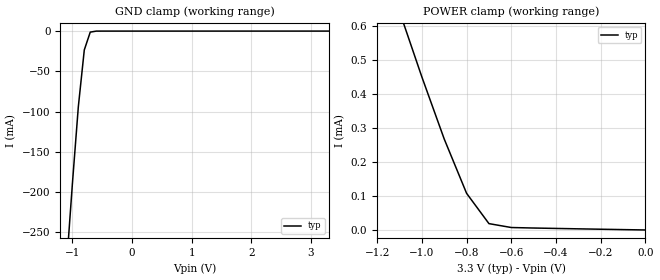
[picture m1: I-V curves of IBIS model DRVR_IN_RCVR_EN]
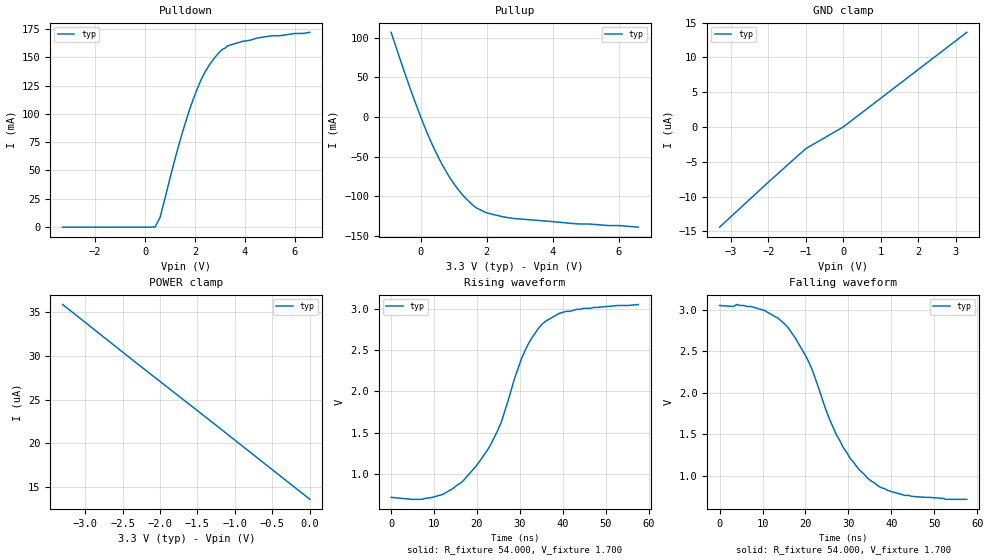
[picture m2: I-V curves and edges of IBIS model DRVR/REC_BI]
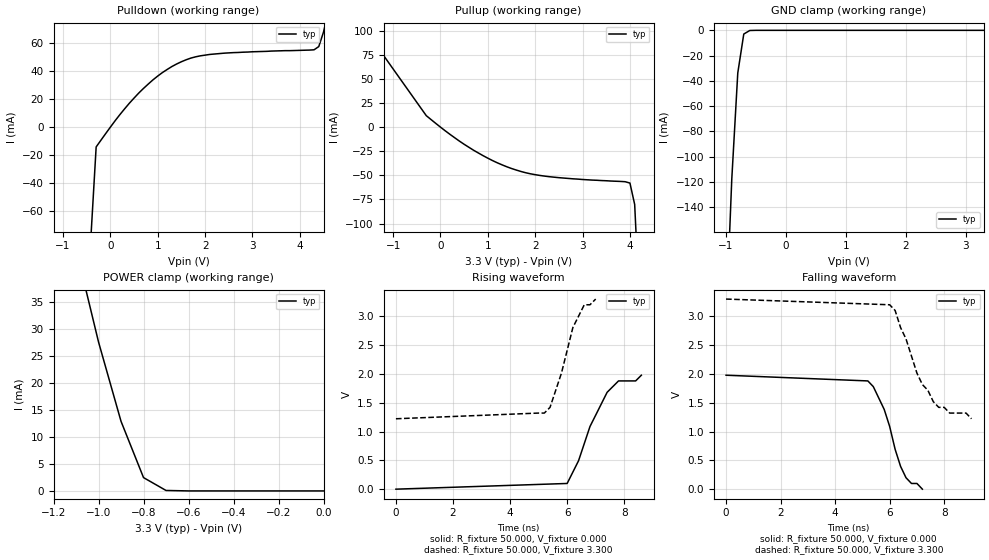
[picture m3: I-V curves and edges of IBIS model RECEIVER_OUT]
|   Texas Instruments Incorporated
|   Data Transmissions Products
|   IBIS Model for SN65HVD11
|   8D SOIC Package
[IBIS Ver]   3.2
[Comment char]   |_char
[File name]   3hvd11.ibs
[File Rev]   1.1
[Date]   11Apr07
[Source]   File originated at Texas Instruments Incorporated.
   Data Transmission Products Group.
[Notes]
[Disclaimer]
(C) Copyright Texas Instruments Incorporated 2002
   All rights reserved
  Texas Instruments Incorporated hereby grants 1the user of this IBIS
model a non-exclusive, nontransferable license to use this IBIS model
under the following terms.  Before using this IBIS model, the user
should read this license.  If the user does not accept these terms,
the IBIS model should be returned to Texas Instruments within 30 days.
  The user is granted this license only to use the IBIS model and
is not granted rights to sell, load, rent, lease or license the IBIS
model in whole or in part, or in modified form to anyone other than
user.  User may modify the IBIS model to suit its specific applications
but rights to derivative works and such modifications shall belong to
Texas Instruments.
  This IBIS model is provided on an "AS IS" basis and Texas Instruments
makes absolutely no warranty with respect to the information contained
herein.  TEXAS INSTRUMENTS DISCLAIMS AND CUSTOMER WAIVES ALL WARRANTIES,
EXPRESS OR IMPLIED, INCLUDING WARRANTIES OF MERCHANTABILITY OR FITNESS
FOR A PARTICULAR PURPOSE. The entire risk as to quality and performance
is with the Customer. ACCORDINGLY, IN NO EVENT SHALL THE COMPANY BE LIABLE
FOR ANY DAMAGES, WHETHER IN CONTRACT OR TORT,INCLUDING ANY LOST PROFITS
OR OTHER INCIDENTAL, CONSEQUENTIAL, EXEMPLARY, OR PUNITIVE DAMAGES ARISING
OUT OF THE USE OR APPLICATION OF THE IBIS model provided in this package.
Further, Texas Instruments reserves the right to discontinue or make changes
without notice to any product herein to improve reliability, function, or
design. Texas Instruments does not convey any license under patent rights
or any other intellectual property rights, including those of third parties.
Contact Texas Instruments at ATTN:DATA TRANSMISSIONS
[Copyright]   Copyright 2002, Texas Instruments, All Rights Reserved
[Component]   HVD11D
[Manufacturer]  Texas Instruments Incorporated
[Package]
|   typ   min   max
R_pkg   0.036   0.033   0.039
L_pkg   3.340nH   2.445nH   4.233nH
C_pkg   0.470pF   0.308pF   0.631pF
[Pin]   signal_name   model_name   R_pin   L_pin   C_pin
1   R   RECEIVER_OUT   0.034   4.233n   0.630p
2   RE   DRVR_IN_RCVR_EN   0.038   2.445n   0.309p
3   DE   DRIVER_EN   0.039   2.448n   0.309p
4   D   DRVR_IN_RCVR_EN   0.033   4.231n   0.631p
5   GND   GND   0.033   4.230n   0.630p
6   A   DRVR/REC_BI   0.039   2.450n   0.308p
7   B   DRVR/REC_BI   0.039   2.448n   0.309p
8   VCC   POWER   0.033   4.231n   0.630p
[Diff_pin]   inv_pin   vdiff   tdelay_typ   tdelay_min   tdelay_max
| The 'A' pin is Diff_pin and the 'B' pin is the inv_pin
6   7   0.200   0 0 0
| Models and submodels in the file (4): DRVR_IN_RCVR_EN (Input), DRIVER_EN (Input), DRVR/REC_BI (I/O), RECEIVER_OUT (3-state)
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|   Driver Input / Receiver Enable Model
[Model]   DRVR_IN_RCVR_EN
Model_type   Input
|Signals   D,RE
Vinh = 2.0
Vinl = 0.8
|   typ   min   max
C_comp   13pF   8pF   16pF
|   typ   min   max
[Temperature Range]   25.0   NA   NA
[Voltage range]   3.3V   3.0V   3.6V
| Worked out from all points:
|   GND clamp passes 1 mA (typ) near -0.68 V on its own axis
|   POWER clamp passes 1 mA (typ) near -1.28 V on its own axis
[GND_clamp]
|   Voltage   I(typ)   I(min)   I(max)
-3.3V     -2.53A     NA         NA
-2V       -1.22A     NA         NA
-1V       -190mA     NA         NA
-900mV    -93.9mA    NA         NA
-800mV    -23.4mA    NA         NA
-700mV    -1.29mA    NA         NA
-600mV    -39.4uA    NA         NA
3.3V      8.15pA     NA         NA
[Power_clamp]
| Note that the[POWER_clamp]voltage table is referenced to Vcc
| and is calculated using Vtable=Vcc - Vmeasured.
|   Voltage   I(typ)   I(min)   I(max)
-3.3V     5.2mA      NA         NA
-1.1V     644uA      NA         NA
-1V       451uA      NA         NA
-900mV    268uA      NA         NA
-800mV    108uA      NA         NA
-700mV    18.7uA     NA         NA
-600mV    7.22uA     NA         NA
0V        8.15pA     NA         NA
|   Driver Output / Receiver Input Model
[Model]   DRVR/REC_BI
Model_type   I/O
| Signals   A,B
Vinl = 0.9V
Vinh = 2.8V
Vmeas = 1.7V   |Reference voltage for timing measurements
Cref = 50pF   |Timing specification test load capacitance value
Rref = 54   |Note: 54 Ohm load; single-ended configuration
|   Timing specification test load voltage
| variable   typ   min   max
C_comp   32pF   26pF   38pF
|   typ   min   max
[Temperature Range]   25.0   NA   NA
[Voltage range]   3.3V   3.0V   3.6V
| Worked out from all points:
|   slope of the pulldown table from 0 to 0.495 V, typ, clamps not added: 120 ohm
|   slope of the pullup table from 0 to 0.495 V, typ, clamps not added: 10.4 ohm
|   rising waveform, R_fixture 54.000, V_fixture 1.700: 20-80 % time 11.1ns typ, NA min, NA max; typ from 0.714 V to 3.05 V
|   falling waveform, R_fixture 54.000, V_fixture 1.700: 20-80 % time 12.4ns typ, NA min, NA max; typ from 3.05 V to 0.714 V
[Pulldown]
|   Voltage   I(typ)   I(min)   I(max)
-3.3V     -26.2uA    NA         NA
400mV     110uA      NA         NA
600mV     8.53mA     NA         NA
1.2V      60.3mA     NA         NA
1.8V      105mA      NA         NA
2.2V      128mA      NA         NA
2.4V      137mA      NA         NA
2.8V      150mA      NA         NA
3.3V      160mA      NA         NA
3.9V      164mA      NA         NA
5.1V      169mA      NA         NA
6.6V      172mA      NA         NA
[Pullup]
|   Voltage   I(typ)   I(min)   I(max)
| Note that the[Pullup]voltage table is referenced to Vcc
| and is calculated using Vtable=Vcc - Vmeasured.
-900mV    107mA      NA         NA
-500mV    57.3mA     NA         NA
-100mV    10.9mA     NA         NA
200mV     -20.7mA    NA         NA
400mV     -39.4mA    NA         NA
700mV     -63.8mA    NA         NA
1V        -83.9mA    NA         NA
1.3V      -99.8mA    NA         NA
1.6V      -112mA     NA         NA
2V        -121mA     NA         NA
2.8V      -128mA     NA         NA
6.6V      -139mA     NA         NA
[GND_clamp]
|   Voltage   I(typ)   I(min)   I(max)
| Outputs in High Impedance (off)
-3.3V     -14.4uA    NA         NA
-2V       -7.94uA    NA         NA
-1V       -3.12uA    NA         NA
0V        -410pA     NA         NA
3.3V      13.6uA     NA         NA
[POWER_clamp]
|   Voltage   I(typ)   I(min)   I(max)
| Note that the [POWER_clamp] voltage table is referenced to Vcc
| and is calculated using Vtable = Vcc - Vmeasured.
| Outputs in Tri-state.
-3.3V     35.9uA     NA         NA
-2.3V     29.1uA     NA         NA
-1.3V     22.4uA     NA         NA
0V        13.6uA     NA         NA
[Ramp]
|   typ   min   max
dV/dt_r   1.188/11.2ns   NA   NA
dV/dt_f   1.200/12.8ns   NA   NA
R_load = 54ohm | Note: The measurement is on a single-ended configuration
|   with 54ohm line-to-line.
[Rising Waveform]
R_fixture = 54.000
V_fixture = 1.700
C_fixture = 0.000
L_fixture = 0.000
|  time   V(typ)   V(min)   V(max)
0s        714mV      NA         NA
7.2ns     690.2mV    NA         NA
12ns      749.6mV    NA         NA
19.2ns    1.058V     NA         NA
22.4ns    1.284V     NA         NA
25.6ns    1.617V     NA         NA
31.2ns    2.496V     NA         NA
36ns      2.852V     NA         NA
43.2ns    2.995V     NA         NA
57.6ns    3.054V     NA         NA
[Falling Waveform]
R_fixture = 54.000
V_fixture = 1.700
C_fixture = 0.000
L_fixture = 0.000
|  time   V(typ)   V(min)   V(max)
0s        3.054V     NA         NA
10.4ns    2.995V     NA         NA
16ns      2.782V     NA         NA
20.8ns    2.369V     NA         NA
25.6ns    1.683V     NA         NA
28.8ns    1.34V      NA         NA
32ns      1.104V     NA         NA
35.2ns    938.6mV    NA         NA
43.2ns    761.3mV    NA         NA
57.6ns    714mV      NA         NA
[Model]   RECEIVER_OUT
Model_type   3-state
| Signals   R
Vmeas = 1.5V   |Reference voltage for timing measurements
Cref = 15pF   |Timing specification test load capacitance value
Vref = 0   |Timing specification test load voltage; GND
| variable   typ   min   max
C_comp   13pF   8pF   16pF
|   typ   min   max
[Temperature Range]   25.0   NA   NA
[Voltage range]   3.3V   3.0V   3.6V
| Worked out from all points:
|   slope of the pulldown table from 0 to 0.495 V, typ, clamps not added: 24.1 ohm
|   slope of the pullup table from 0 to 0.495 V, typ, clamps not added: 28.1 ohm
|   GND clamp passes 1 mA (typ) near -0.63 V on its own axis
|   POWER clamp passes 1 mA (typ) near -0.74 V on its own axis
|   rising waveform, R_fixture 50.000, V_fixture 0.000: 20-80 % time 1ns typ, NA min, NA max; typ from 0 V to 1.98 V
|   falling waveform, R_fixture 50.000, V_fixture 0.000: 20-80 % time 800ps typ, NA min, NA max; typ from 1.98 V to 0 V
|   rising waveform, R_fixture 50.000, V_fixture 3.300: 20-80 % time 734ps typ, NA min, NA max; typ from 1.22 V to 3.3 V
|   falling waveform, R_fixture 50.000, V_fixture 3.300: 20-80 % time 1.13ns typ, NA min, NA max; typ from 3.3 V to 1.22 V
[Pulldown]
|   Voltage   I(typ)   I(min)   I(max)
-3.3V     -2.97A     NA         NA
-1.3V     -595mA     NA         NA
-300mV    -14.1mA    NA         NA
200mV     8.88mA     NA         NA
900mV     33.7mA     NA         NA
1.5V      46.6mA     NA         NA
2.1V      51.8mA     NA         NA
4.3V      55.1mA     NA         NA
4.4V      57.4mA     NA         NA
4.5V      67.7mA     NA         NA
4.6V      82.3mA     NA         NA
6.6V      434mA      NA         NA
[Pullup]
|   Voltage   I(typ)   I(min)   I(max)
| Note that the[Pullup]voltage table is referenced to Vcc
| and is calculated using Vtable=Vcc - Vmeasured.
-3.3V     434mA      NA         NA
-2.3V     255mA      NA         NA
-1.3V     81.1mA     NA         NA
-300mV    11.9mA     NA         NA
500mV     -17.8mA    NA         NA
1.2V      -37mA      NA         NA
1.7V      -46mA      NA         NA
2.1V      -50.1mA    NA         NA
4V        -58mA      NA         NA
4.1V      -80.2mA    NA         NA
4.6V      -596mA     NA         NA
6.6V      -2.97A     NA         NA
[GND_clamp]
|   Voltage   I(typ)   I(min)   I(max)
| Outputs in High Impedance (off)
-3.3V     -2.97A     NA         NA
-1.3V     -591mA     NA         NA
-900mV    -118mA     NA         NA
-800mV    -33.8mA    NA         NA
-700mV    -2.94mA    NA         NA
-600mV    -137uA     NA         NA
3.3V      43.8pA     NA         NA
[POWER_clamp]
|   Voltage   I(typ)   I(min)   I(max)
| Note that the [POWER_clamp] voltage table is referenced to Vcc
| and is calculated using Vtable = Vcc - Vmeasured.
| Outputs in Tri-state.
-3.3V     434mA      NA         NA
-2V       200mA      NA         NA
-1V       27.6mA     NA         NA
-900mV    12.9mA     NA         NA
-800mV    2.47mA     NA         NA
-700mV    85.2uA     NA         NA
-600mV    1.82uA     NA         NA
-500mV    38.6nA     NA         NA
-400mV    871pA      NA         NA
-300mV    68.6pA     NA         NA
0V        43.8pA     NA         NA
[Ramp]
|   typ   min   max
dV/dt_r   2.71V/2.16ns   NA   NA
dV/dt_f   2.55V/3.15ps   NA   NA
R_load = 50
[Rising Waveform]
R_fixture = 50.000
V_fixture = 0.000
C_fixture = 0.000
L_fixture = 0.000
|  time   V(typ)   V(min)   V(max)
0s        4.483nV    NA         NA
6ns       98.88mV    NA         NA
6.4ns     494.4mV    NA         NA
6.8ns     1.088V     NA         NA
7.4ns     1.681V     NA         NA
7.8ns     1.879V     NA         NA
8.4ns     1.879V     NA         NA
8.6ns     1.978V     NA         NA
[Falling Waveform]
R_fixture = 50.000
V_fixture = 0.000
C_fixture = 0.000
L_fixture = 0.000
|  time   V(typ)   V(min)   V(max)
0s        1.978V     NA         NA
5.2ns     1.879V     NA         NA
5.4ns     1.78V      NA         NA
5.8ns     1.384V     NA         NA
6ns       1.088V     NA         NA
6.2ns     692.1mV    NA         NA
6.4ns     395.5mV    NA         NA
6.6ns     197.8mV    NA         NA
6.8ns     98.88mV    NA         NA
7.2ns     4.483nV    NA         NA
[Rising Waveform]
R_fixture = 50.000
V_fixture = 3.300
C_fixture = 0.000
L_fixture = 0.000
|  time   V(typ)   V(min)   V(max)
0s        1.222V     NA         NA
5.2ns     1.321V     NA         NA
5.4ns     1.42V      NA         NA
5.8ns     2.014V     NA         NA
6.2ns     2.805V     NA         NA
6.6ns     3.201V     NA         NA
6.8ns     3.201V     NA         NA
7ns       3.3V       NA         NA
[Falling Waveform]
R_fixture = 50.000
V_fixture = 3.300
C_fixture = 0.000
L_fixture = 0.000
|  time   V(typ)   V(min)   V(max)
0s        3.3V       NA         NA
6ns       3.201V     NA         NA
6.2ns     3.102V     NA         NA
6.4ns     2.805V     NA         NA
6.6ns     2.607V     NA         NA
7ns       2.014V     NA         NA
7.6ns     1.519V     NA         NA
8.2ns     1.321V     NA         NA
8.8ns     1.321V     NA         NA
9ns       1.222V     NA         NA
